(* Logix 5000 Rung export; software revision 20.05 *)

TYPE ProSoftHARTDiagnostics :
STRUCT
   DeviceSpecificStatus0_0 : SINT;
   DeviceSpecificStatus0_1 : SINT;
   DeviceSpecificStatus0_2 : SINT;
   DeviceSpecificStatus0_3 : SINT;
   DeviceSpecificStatus0_4 : SINT;
   DeviceSpecificStatus0_5 : SINT;
   Reserved0 : SINT;
   Reserved1 : SINT;
   OperationMode_0 : SINT;
   OperationMode_1 : SINT;
   Reserved2 : SINT;
   Reserved3 : SINT;
   StandardizedStatus0 : SINT;
   StandardizedStatus1 : SINT;
   AnalogChannelSaturated : SINT;
   StandardizedStatus2 : SINT;
   StandardizedStatus3 : SINT;
   AnalogChannelFixed : SINT;
   DeviceSpecific1_0 : SINT;
   DeviceSpecific1_1 : SINT;
   DeviceSpecific1_2 : SINT;
   DeviceSpecific1_3 : SINT;
   DeviceSpecific1_4 : SINT;
   DeviceSpecific1_5 : SINT;
   DeviceSpecific1_6 : SINT;
   DeviceSpecific1_7 : SINT;
   DeviceSpecific1_8 : SINT;
   DeviceSpecific1_9 : SINT;
   DeviceSpecific1_10 : SINT;
END_STRUCT
END_TYPE

TYPE ProSoftHARTStatus :
STRUCT
   ParityError : BOOL;
   OverrunError : BOOL;
   FramingError : BOOL;
   ChecksumError : BOOL;
   RxBufferOverflow : BOOL;
   ValueTooLarge : BOOL;
   ValueTooSmall : BOOL;
   NotEnoughBytesInCommand : BOOL;
   TransmitterSpecificCmdError : BOOL;
   InWriteProtectMode : BOOL;
   UpdateFailed : BOOL;
   AppliedProcessTooHigh : BOOL;
   AppliedProcessTooLow : BOOL;
   InMultidropMode : BOOL;
   InvalidUnitCode : BOOL;
   BothRangeValuesOutOfLimits : BOOL;
   PushedUpperRangeValueOverLimit : BOOL;
   AccessRestricted : BOOL;
   DeviceBusy : BOOL;
   CommandNotImplemented : BOOL;
   DeviceMalfunction : BOOL;
   ConfigurationChanged : BOOL;
   Coldstart : BOOL;
   MoreStatusAvailable : BOOL;
   LoopCurrentFixed : BOOL;
   LoopCurrentSaturated : BOOL;
   NonPrimaryVariableOutOFLimits : BOOL;
   PrimaryVariableOutOfLimites : BOOL;
END_STRUCT
END_TYPE

TYPE ProSoftHARTRelayMessageResponse :
STRUCT
   Status : INT;
   PacketLength : INT;
   StartCharacter : SINT;
   AddressByte0 : SINT;
   AddressByte1 : SINT;
   AddressByte2 : SINT;
   AddressByte3 : SINT;
   AddressByte4 : SINT;
   Command : SINT;
   ByteCount : SINT;
   Data : SINT[50];
END_STRUCT
END_TYPE

TYPE Input :
STRUCT
   FixAddrData : ProSoftHART4Input;
END_STRUCT
END_TYPE

TYPE ProSoftHARTMultidropLegacy :
STRUCT
   Auto_Poll_CMD_Status : SINT;   // Auto-Polling command status bits
   Last_Status_Byte : SINT;   // Last first status byte received from device
   Last_Second_Status_Byte : SINT;   // Last second status byte received from device
   Manufacture_ID_Code : SINT;   // Device's Manufacture ID Code
   Device_Type_Code : SINT;   // Device Type Code
   Min_Preambles : SINT;   // Minimum Number of Preambles
   Universal_CMD_Major : SINT;   // Universal Command Major Revision Number
   Device_Rev_Level : SINT;   // Device Revision Level
   Software_Rev_Level : SINT;   // Software Revision Level
   Hardware_Rev_Level : SINT;   // Hardware Revision Level
   Device_Flags : SINT;   // Device Flags
   Device_ID : SINT[3];   // Device ID
   Min_Preambles_Resp : SINT;   // Minimum Preambles Count to Response
   Max_Number_Devices : SINT;   // Maximum Number of HART Devices in the Network
   Config_Change_Count : INT;   // Counter for Configuration Changes
   Ext_Dev_Status : SINT;   // Extended Field Device Status
   Primary_Var_Units : SINT;   // Primary Units Code
   Secondary_Var_Units : SINT;   // Secondary Units Code
   Tertiary_Var_Units : SINT;   // Tertiary Units Code
   Quaternary_Var_Units : SINT;   // Quaternary Units Code
   Tag_Name : SINT[8];   // HART Device Tag Name
   Descriptor : SINT[16];   // HART Device Descriptor
   Tag_Descriptor_Date : SINT[3];   // HART Device Descriptor Date
   Transd_Serial_Num : SINT[3];   // Transducer Serial Number
   Transd_limits : SINT;   // Transducer Limits
   PV_Alarms : SINT;   // PV Alarm Counter
   PV_Transfer : SINT;   // PV Transfer Counter
   PV_URLLRV_Units : SINT;   // PV Upper and Lower Value Limits
   Write_Protection_Code : SINT;   // Write Protection Code
   Private_Label_Code : SINT;   // Private Label Distributor Code
   PV_Analog_Ch_Flag : SINT;   // PV Analog Channel Flag
   PV_value : REAL;   // Primary Variable Value
   SV_value : REAL;   // Secondary Variable Value
   TV_value : REAL;   // Tertiary Variable Value
   QV_value : REAL;   // Quaternary Variable Value
   U_trans_limit : REAL;   // Upper Transducer Limit
   L_trans_limit : REAL;   // Lower Transducer Limit
   Min_span : REAL;   // Minimum Span
   PV_URV : REAL;   // PV Upper Range Value
   PV_LRV : REAL;   // PV Lower Range Value
   PV_damp : REAL;   // PV Damping Value
END_STRUCT
END_TYPE

TYPE ProSoftHARTMultidrop :
STRUCT
   PollStatus : SINT;   // Auto-Polling command status bits
   LastStatusByte : SINT;   // Last first status byte received from device
   LastSecond_StatusByte : SINT;   // Last second status byte received from device
   ManufactureIDCode : SINT;   // Device's Manufacture ID Code
   DeviceTypeCode : SINT;   // Device Type Code
   MinPreambles : SINT;   // Minimum Number of Preambles
   UniversalCMDMajor : SINT;   // Universal Command Major Revision Number
   DeviceRevision : SINT;   // Device Revision Level
   SoftwareRevision : SINT;   // Software Revision Level
   HardwareRevision : SINT;   // Hardware Revision Level
   DeviceFlags : SINT;   // Device Flags
   DeviceID : DINT;   // Device ID
   PreambleResponse : SINT;   // Minimum Preambles Count to Response
   MaxNumberDeviceVariables : SINT;   // Maximum Number of HART Device Variables
   ConfigChangeCount : INT;   // Counter for Configuration Changes
   ExtDeviceStatus : SINT;   // Extended Field Device Status
   PVUnits : SINT;   // Primary Units Code
   SVUnits : SINT;   // Secondary Units Code
   TVUnits : SINT;   // Tertiary Units Code
   FVUnits : SINT;   // Quaternary Units Code
   Tagname : ProsoftSTRING8;   // HART Device Tag Name
   Descriptor : ProsoftSTRING16;   // HART Device Descriptor
   TagDescriptorDate : ProsoftSTRING8;   // HART Device Descriptor Date
   SerialNumber : DINT;   // Transducer Serial Number
   TransducerLimits : SINT;   // Transducer Limits
   PVAlarms : SINT;   // PV Alarm Counter
   PVTransfer : SINT;   // PV Transfer Counter
   PVURLLRV_Units : SINT;   // PV Upper and Lower Value Limits
   WriteProtectionCode : SINT;   // Write Protection Code
   PrivateLabelCode : SINT;   // Private Label Distributor Code
   PVAnalogChFlag : SINT;   // PV Analog Channel Flag
   PV : REAL;   // Primary Variable Value
   SV : REAL;   // Secondary Variable Value
   TV : REAL;   // Tertiary Variable Value
   FV : REAL;   // Quaternary Variable Value
   UpperTransducerLimit : REAL;   // Upper Transducer Limit
   LowerTransducerLimit : REAL;   // Lower Transducer Limit
   MinimumSpan : REAL;   // Minimum Span
   PVUpperRange : REAL;   // PV Upper Range Value
   PVLowerRange : REAL;   // PV Lower Range Value
   PVDamping : REAL;   // PV Damping Value
END_STRUCT
END_TYPE

TYPE ProSoftStatus :
STRUCT
   PLX51Status : ProSoftHARTModuleStatus;
   HartStatus : ProSoftHARTStatus;
   DeviceStatus : ProSoftHARTDeviceStatus;
   DeviceDiagnostics : ProSoftHARTDiagnostics;
END_STRUCT
END_TYPE

TYPE ProSoftHARTDeviceStatus :
STRUCT
   LoopOpen : BOOL;
   CurrentUnderrange : BOOL;
   CurrentOverrange : BOOL;
   LoopShorted : BOOL;
   CalibrationBusy : BOOL;
   CalibrationFaulted : BOOL;
   HARTCommsFault : BOOL;
   RelayMessagesInhibited : BOOL;
END_STRUCT
END_TYPE

TYPE PLX51HART4I :
STRUCT
   Input : Input;
   Control : MessageControl;
   Status : ProSoftStatus;
   MultiDropCH0 : ProSoftHARTMultidrop[7];
   MultiDropCH1 : ProSoftHARTMultidrop[7];
   MultiDropCH2 : ProSoftHARTMultidrop[7];
   MultiDropCH3 : ProSoftHARTMultidrop[7];
   LegacyPolling : ProSoftHARTMultidropLegacy[5];
END_STRUCT
END_TYPE

TYPE ProSoftHART4Input :
STRUCT
   Instance : ProsoftSTRING16;
   Status : ProSoftHARTModuleStatus;
   Temperature : REAL;
   Ch0_ManufacturerID : SINT;
   Ch0_ManufacturerDeviceType : SINT;
   Ch0_DeviceID : DINT;
   Ch0_Tag : ProsoftSTRING8;
   Ch0_Descriptor : ProsoftSTRING16;
   Ch0_DeviceStatus : ProSoftHARTDeviceStatus;
   Ch0_HARTStatus : ProSoftHARTStatus;
   Ch0_RawCurrent : REAL;
   Ch0_ScaledValue : REAL;
   Ch0_DigitialCurrent : REAL;
   Ch0_PV : REAL;
   Ch0_SV : REAL;
   Ch0_TV : REAL;
   Ch0_FV : REAL;
   Ch0_PVUnitCode : SINT;
   Ch0_SVUnitCode : SINT;
   Ch0_TVUnitCode : SINT;
   Ch0_FVUnitCode : SINT;
   Ch0_Diagnostics : ProSoftHARTDiagnostics;
   Ch1_ManufacturerID : SINT;
   Ch1_ManufacturerDeviceType : SINT;
   Ch1_DeviceID : DINT;
   Ch1_Tag : ProsoftSTRING8;
   Ch1_Descriptor : ProsoftSTRING16;
   Ch1_DeviceStatus : ProSoftHARTDeviceStatus;
   Ch1_HARTStatus : ProSoftHARTStatus;
   Ch1_RawCurrent : REAL;
   Ch1_ScaledValue : REAL;
   Ch1_DigitialCurrent : REAL;
   Ch1_PV : REAL;
   Ch1_SV : REAL;
   Ch1_TV : REAL;
   Ch1_FV : REAL;
   Ch1_PVUnitCode : SINT;
   Ch1_SVUnitCode : SINT;
   Ch1_TVUnitCode : SINT;
   Ch1_FVUnitCode : SINT;
   Ch1_Diagnostics : ProSoftHARTDiagnostics;
   Ch2_ManufacturerID : SINT;
   Ch2_ManufacturerDeviceType : SINT;
   Ch2_DeviceID : DINT;
   Ch2_Tag : ProsoftSTRING8;
   Ch2_Descriptor : ProsoftSTRING16;
   Ch2_DeviceStatus : ProSoftHARTDeviceStatus;
   Ch2_HARTStatus : ProSoftHARTStatus;
   Ch2_RawCurrent : REAL;
   Ch2_ScaledValue : REAL;
   Ch2_DigitialCurrent : REAL;
   Ch2_PV : REAL;
   Ch2_SV : REAL;
   Ch2_TV : REAL;
   Ch2_FV : REAL;
   Ch2_PVUnitCode : SINT;
   Ch2_SVUnitCode : SINT;
   Ch2_TVUnitCode : SINT;
   Ch2_FVUnitCode : SINT;
   Ch2_Diagnostics : ProSoftHARTDiagnostics;
   Ch3_ManufacturerID : SINT;
   Ch3_ManufacturerDeviceType : SINT;
   Ch3_DeviceID : DINT;
   Ch3_Tag : ProsoftSTRING8;
   Ch3_Descriptor : ProsoftSTRING16;
   Ch3_DeviceStatus : ProSoftHARTDeviceStatus;
   Ch3_HARTStatus : ProSoftHARTStatus;
   Ch3_RawCurrent : REAL;
   Ch3_ScaledValue : REAL;
   Ch3_DigitialCurrent : REAL;
   Ch3_PV : REAL;
   Ch3_SV : REAL;
   Ch3_TV : REAL;
   Ch3_FV : REAL;
   Ch3_PVUnitCode : SINT;
   Ch3_SVUnitCode : SINT;
   Ch3_TVUnitCode : SINT;
   Ch3_FVUnitCode : SINT;
   Ch3_Diagnostics : ProSoftHARTDiagnostics;
END_STRUCT
END_TYPE

TYPE ProSoftHARTModuleStatus :
STRUCT
   ConfigurationValid : BOOL;
   Channel0Enabled : BOOL;
   Channel1Enabled : BOOL;
   Channel2Enabled : BOOL;
   Channel3Enabled : BOOL;
   Channel0HARTEnabled : BOOL;
   Channel1HARTEnabled : BOOL;
   Channel2HARTEnabled : BOOL;
   Channel3HARTEnabled : BOOL;
END_STRUCT
END_TYPE

TYPE ProSoftHARTRelayMessageRequest :
STRUCT
   Length : INT;
   StartCharacter : SINT;
   AddressByte0 : SINT;
   AddressByte1 : SINT;
   AddressByte2 : SINT;
   AddressByte3 : SINT;
   AddressByte4 : SINT;
   CommandData : SINT[40];
END_STRUCT
END_TYPE

TYPE ProsoftSTRING8 :   // string type
STRUCT
   LEN : DINT;
   DATA : SINT[8];
END_STRUCT
END_TYPE

TYPE MessageControl :
STRUCT
   TriggerMessage : BOOL;
   MessageRequest : ProSoftHARTRelayMessageRequest;
   MessageResponse : ProSoftHARTRelayMessageResponse;
END_STRUCT
END_TYPE

TYPE ProsoftSTRING16 :   // string type
STRUCT
   LEN : DINT;
   DATA : SINT[16];
END_STRUCT
END_TYPE

VAR_GLOBAL   (* controller tags *)
   HARTMessage : MESSAGE;
        MessageParameters(MessageType := CIP Generic, RequestedLength := 48, ConnectedFlag := 2, ConnectionPath := PLX51HART4I, ServiceCode := 16#0079, ObjectType := 16#040f, TargetObject := 1, LocalElement := PLX51HART4IN.Control.MessageRequest, DestinationTag := PLX51HART4IN.Control.MessageResponse)
   PLX51HART4I:I : AB:ETHERNET_MODULE_DINT_476Bytes:I:0 := (Data[0] := 10, Data[1] := 1953653064, Data[2] := 1852403536, Data[3] := 13172, Data[5] := 1, Data[6] := 1112120821, Data[7] := 14353, Data[8] := 16732025, Data[9] := 8, Data[10] := 808539206, Data[11] := 538976310, Data[12] := 16, Data[13] := 1397899597, Data[14] := 538976328, Data[15] := 538976288, Data[16] := 538976288, Data[17] := 67, Data[18] := 2097152, Data[19] := 1052566482, Data[20] := 1072438470, Data[21] := 1082130432, Data[26] := 724257555, Data[35] := 14353, Data[36] := 16732025, Data[37] := 8, Data[38] := 808539206, Data[39] := 538976310, Data[40] := 16, Data[41] := 1397899597, Data[42] := 538976328, Data[43] := 538976288, Data[44] := 538976288, Data[46] := 2097152, Data[47] := 1081730770, Data[48] := 1093226191, Data[49] := 1082130432, Data[54] := 724257555, Data[73] := 64, Data[101] := 64);
   PLX51HART4IN : PLX51HART4I;
END_VAR

PROGRAM MainProgram

ROUTINE HART4I_Routine   (* ladder *)
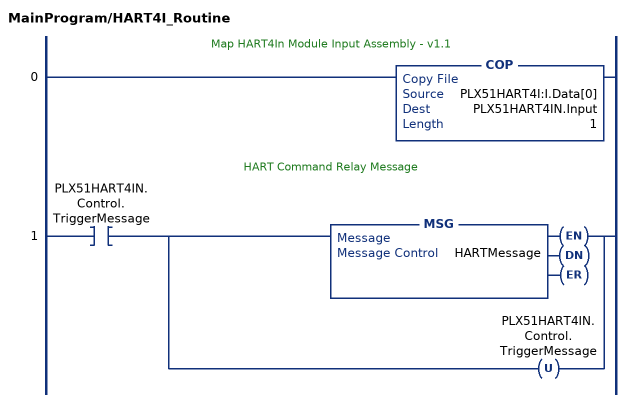
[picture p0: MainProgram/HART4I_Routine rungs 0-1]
   // Map HART4In Module Input Assembly - v1.1
   0: COP(PLX51HART4I:I.Data[0],PLX51HART4IN.Input,1);
   // HART Command Relay Message
   1: XIC(PLX51HART4IN.Control.TriggerMessage)[MSG(HARTMessage) ,OTU(PLX51HART4IN.Control.TriggerMessage) ];
END_ROUTINE
END_PROGRAM
